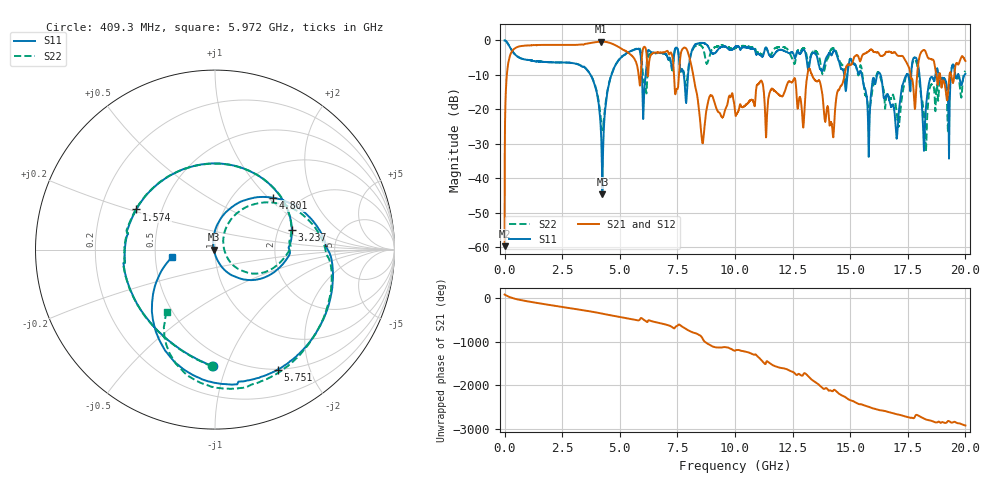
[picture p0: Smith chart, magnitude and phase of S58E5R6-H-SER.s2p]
!{S58E5R6}
!Johanson Technology Inc.
!www.johansontechnology.com
!Test Board Conditions:
!Substrate Type  RO4350B
!Substrate Thickness  60 mil
!Substrate Dk  3.66
!TL Type: GCPW
!TL Trace Width  115 mil
!TL Gap  52 mil
!Electrode orientation  Horizontal
!DUT TOPOLOGY	SERIES
!Mounting Pad LxW  55x428 mil
! Created Tue Apr 13 22:41:05 2021
# hz S ma R 50
! 2 Port Network Data from SP1.SP block
! freq  magS11  angS11  magS21  angS21  magS12  angS12  magS22  angS22
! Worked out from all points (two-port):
!   20001 points, 300 kHz to 20 GHz, reference 50 ohm
!   highest |S21| = -0.32 dB at 4.193 GHz (marker M1); lowest = -59.7 dB at 300 kHz (marker M2)
!   |S21| within 3 dB of the highest: 305.4 MHz to 5.315 GHz (5.009 GHz wide, 178 % of centre); 7.664 GHz to 7.95 GHz (286.4 MHz wide, 3.67 % of centre)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
!   lowest |S11| = -44.7 dB at 4.244 GHz (marker M3), VSWR 1.01, Z = 49.4 - j0.0261 ohm
!   |S11| at or under -10 dB: 3.73 GHz to 4.635 GHz (904.8 MHz wide, 21.6 % of centre); 16.32 GHz to 17.44 GHz (1.116 GHz wide, 6.61 % of centre); 18.01 GHz to 18.7 GHz (690.8 MHz wide, 3.76 % of centre)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
!   |S22| runs from -32.2 to 0.0 dB; largest |S21 - S12| = 0.017
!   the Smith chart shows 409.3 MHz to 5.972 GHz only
!   S11 on the Smith chart (normalised r, x): 409.3 MHz: 0.40, -0.90; 1.574 GHz: 0.36, +0.21; 3.237 GHz: 2.38, +0.64; 4.801 GHz: 1.49, +1.06; 5.751 GHz: 0.50, -1.54; 5.972 GHz: 0.62, -0.05
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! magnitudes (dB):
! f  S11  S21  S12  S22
! 300 kHz  0.0  -59.7  -60.4  0.0
! 121.3 MHz  -0.7  -8.4  -8.4  -0.7
! 409.3 MHz  -3.8  -2.5  -2.4  -3.7
! 1.574 GHz  -6.1  -1.3  -1.3  -6.1
! 3.237 GHz  -7.1  -1.2  -1.2  -7.0
! 3.334 GHz  -7.4  -1.2  -1.2  -7.4
! 4.193 GHz  -28.0  -0.3  -0.3  -23.9
! 4.244 GHz  -44.7  -0.3  -0.3  -26.0
! 4.801 GHz  -7.3  -1.4  -1.4  -7.2
! 5.751 GHz  -2.4  -7.3  -7.3  -2.3
! 5.972 GHz  -12.4  -3.9  -3.9  -7.3
! 6.667 GHz  -3.7  -3.5  -3.5  -3.7
! 7.906 GHz  -16.1  -2.6  -2.6  -12.1
! 8.587 GHz  -0.7  -29.8  -29.5  -1.9
! 10 GHz  -1.9  -20.7  -20.7  -2.2
! 13.33 GHz  -3.9  -9.9  -9.8  -3.7
! 14.21 GHz  -4.2  -24.7  -24.6  -2.4
! 14.88 GHz  -9.8  -7.0  -7.0  -9.1
! 16.67 GHz  -16.5  -3.2  -3.3  -16.3
! 17.81 GHz  -4.9  -19.9  -19.7  -5.6
! 18.27 GHz  -21.6  -3.2  -3.2  -29.3
! 20 GHz  -9.7  -5.9  -5.9  -8.9
